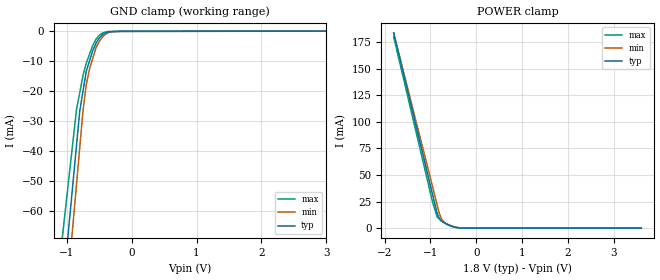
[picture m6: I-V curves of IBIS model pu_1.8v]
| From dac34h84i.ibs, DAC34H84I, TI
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[Model] pu_1.8v
Model_type Input
Vinl = 540.000mV
Vinh = 1.26000V
C_comp 609.000fF 588.000fF 630.000fF
| variable typ   min   max
[Voltage Range] 1.80000V 1.70000V 1.90000V
[POWER Clamp Reference] 1.80000V 1.70000V 1.90000V
[GND Clamp Reference] 0.00000V 0.00000V 0.00000V
[Temperature Range] 25   125   -40
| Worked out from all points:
|   GND clamp passes 1 mA (typ) near -0.44 V on its own axis
|   POWER clamp passes 1 mA (typ) near -0.47 V on its own axis
[GND Clamp]
-1.8V     -255.6mA   -283.5mA   -211.4mA
-850mV    -37.96mA   -50.92mA   -26.01mA
-800mV    -26.51mA   -38.68mA   -20.38mA
-750mV    -19.93mA   -26.44mA   -14.75mA
-700mV    -13.36mA   -17.82mA   -10.62mA
-650mV    -9.903mA   -12.58mA   -7.663mA
-600mV    -6.45mA    -9.058mA   -4.705mA
-550mV    -3.988mA   -5.541mA   -2.687mA
-450mV    -1.123mA   -1.895mA   -584uA
-350mV    -171.7uA   -401.2uA   -62.57uA
-150mV    -14.94uA   -44.13uA   -17.39uA
3.6V      33.51uA    60.01uA    20.56uA
[POWER Clamp]
-1.8V     183.6mA    183.6mA    179.9mA
-950mV    31.27mA    38.65mA    24.14mA
-850mV    13.35mA    21.59mA    10.35mA
-800mV    8.74mA     13.07mA    8.426mA
-750mV    6.43mA     8.077mA    6.503mA
-700mV    5.122mA    5.723mA    5.184mA
-600mV    2.935mA    3.106mA    2.871mA
-450mV    790.2uA    1.058mA    637.6uA
-300mV    107.2uA    102uA      60.97uA
3.6V      0A         0A         0A
